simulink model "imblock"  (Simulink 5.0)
settings: Solver=ode45  StartTime=0.0  StopTime=10.0  RelTol=1e-3
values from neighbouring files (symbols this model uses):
  ic = [fs0 fr0]    [imdef0vec.m]    (also in imdef1vec.m; imdef2vec.m = F; imic2.m = [phids phiqs phidr phiqr n0]'; imic3.m = [phids phiqs phidr phiqr n0]')
libraries: simulink x1

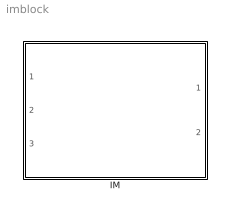
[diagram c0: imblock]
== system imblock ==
  IM : Subsystem  mask{Rs=0.02, Rr=0.01, Lsl=0.1, Lrl=0.1, Lm=5, wo=2*pi*60}
      mask prompts: Rs "Stator resistance [pu]"; Rr "Rotor resistance [pu]"; Lsl "Stator leakage inductance [pu]"; Lrl "Rotor leakage inductance [pu]"; Lm "Magnetizing inductance [pu]"; wo "Base frequency [rad/s]"
      mask help: Induction motor state space model in arbitrary reference frame. Parameters are expressed in per unit.
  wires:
  IM/1(Te) -> ?
  IM/2(is) -> ?
  ? -> IM/1(vs)
  ? -> IM/2(wk)
  ? -> IM/3(wm)

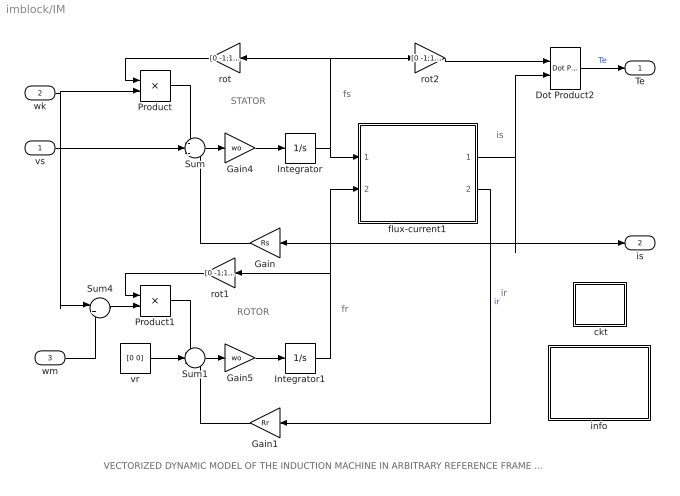
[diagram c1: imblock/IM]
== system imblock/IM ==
  note: ROTOR
  note: STATOR
  note: fs
  note: fr
  note: is
  note: VECTORIZED DYNAMIC MODEL OF THE INDUCTION MACHINE IN ARBITRARY REFERENCE FRAME (per unit formulation)
  note: ir
  vs : Inport
  wk : Inport  Port=2
  wm : Inport  Port=3
  " ckt" : Subsystem
  Dot Product2 : simulink/Math Operations/Dot Product
  Gain : Gain  Orientation=left  Gain=Rs
  Gain1 : Gain  Orientation=left  Gain=Rr
  Gain4 : Gain  Gain=wo
  Gain5 : Gain  Gain=wo
  Integrator : Integrator  InitialCondition=[ic(1) ic(2)]
  Integrator1 : Integrator  InitialCondition=[ic(3) ic(4)]
  Product : Product
  Product1 : Product
  Sum : Sum  Inputs=-+-
  Sum1 : Sum  Inputs=-+-
  Sum4 : Sum  Inputs=|+-
  flux-current1 : Subsystem
  info : Subsystem
  rot : Gain  Orientation=left  Gain=[0 -1;1 0]  Multiplication=Matrix(K*u)
  rot1 : Gain  Orientation=left  Gain=[0 -1;1 0]  Multiplication=Matrix(K*u)
  rot2 : Gain  Gain=[0 -1;1 0]  Multiplication=Matrix(K*u)
  vr : Constant  Value=[0 0]
  Te : Outport
  is : Outport  Port=2
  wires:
  Gain/1 -> Sum/3
  vr/1 -> Sum1/2
  Gain1/1 -> Sum1/3
  flux-current1/2(ir) -> Gain1/1  "ir"
  Integrator/1 -> flux-current1/1(fs), rot/1, rot2/1
  Integrator1/1 -> rot1/1, flux-current1/2(fr)
  Product1/1 -> Sum1/1
  rot1/1 -> Product1/1
  Product/1 -> Sum/1
  rot/1 -> Product/1
  rot2/1 -> Dot Product2/1
  Sum4/1 -> Product1/2
  Sum/1 -> Gain4/1
  Gain4/1 -> Integrator/1
  Sum1/1 -> Gain5/1
  Gain5/1 -> Integrator1/1
  flux-current1/1(is) -> Gain/1, is/1, Dot Product2/2
  Dot Product2/1 -> Te/1  "Te"
  vs/1 -> Sum/2
  wk/1 -> Product/2, Sum4/1
  wm/1 -> Sum4/2

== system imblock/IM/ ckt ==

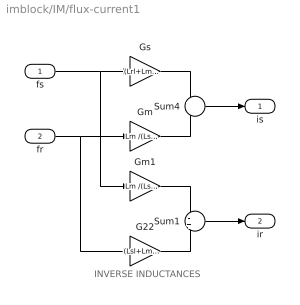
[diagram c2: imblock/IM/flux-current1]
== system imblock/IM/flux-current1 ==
  note: INVERSE INDUCTANCES
  fs : Inport
  fr : Inport  Port=2
  G22 : Gain  Gain=(Lsl+Lm )/(Lsl*Lrl+Lsl*Lm+Lrl*Lm)
  Gm : Gain  Gain=Lm /(Lsl*Lrl+Lsl*Lm+Lrl*Lm)
  Gm1 : Gain  Gain=Lm /(Lsl*Lrl+Lsl*Lm+Lrl*Lm)
  Gs : Gain  Gain=(Lrl+Lm) /(Lsl*Lrl+Lsl*Lm+Lrl*Lm)
  Sum1 : Sum  Inputs=-+
  Sum4 : Sum  Inputs=+-
  is : Outport
  ir : Outport  Port=2
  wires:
  fs/1 -> Gs/1, Gm1/1
  Gs/1 -> Sum4/1
  fr/1 -> Gm/1, G22/1
  Gm/1 -> Sum4/2
  Sum4/1 -> is/1
  Gm1/1 -> Sum1/1
  G22/1 -> Sum1/2
  Sum1/1 -> ir/1

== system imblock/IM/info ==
  note: Mathematical model of the induction machine. Space vector formulation in an arbitrary dq common reference frame. Per unit description.
  note: Electrical system equations: vs = Rs is + 1/wo (dfs/dt) + wk M(pi/2) fs vr = Rr ir + 1/wo (dfr/dt) + (wk - wm) M(pi/2) fr where the variables i, v, and f are 2-dimensional space vectors; for instance is = [ids iqs] and so forth, wk is the speed of the reference frame, wm the rotor speed, and M(pi/2)represents a 90o space rotator namely M(pi/2) = [0 -1;1 0] The flux linkage current relations are: fs = Ls is + Lm ir fr = Lm is + Lr ir where Ls =Lm +Lsl and Lr = Lm +Lrl Mechanical system equations: Te = 2H (dwm/dt ) + Bm wm + Tl where Te = fs (cross) is = M(pi/2) fs (dot) is = fds iqs - fqs ids = fs x is = M(pi/2) fs . is = ir x fr = Lm (ir x is) = Lm/Lr (fr x is) = 1/Lm' (fr x fs) Lm' =Lm c/(1-c) c = 1 - Lm^2/(Ls Lr)
